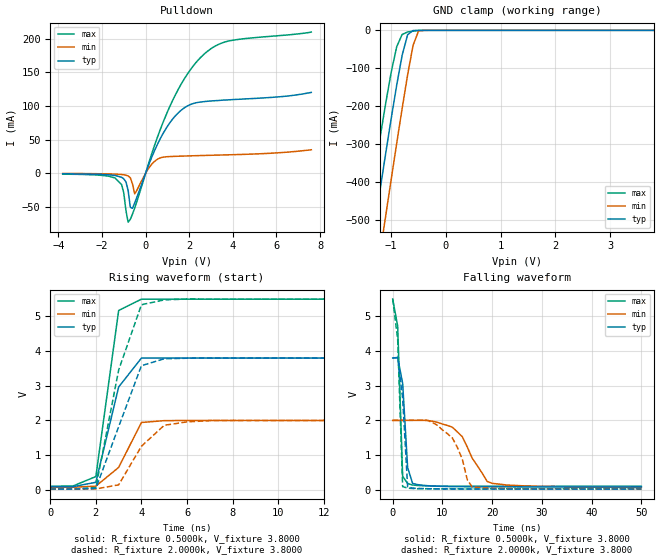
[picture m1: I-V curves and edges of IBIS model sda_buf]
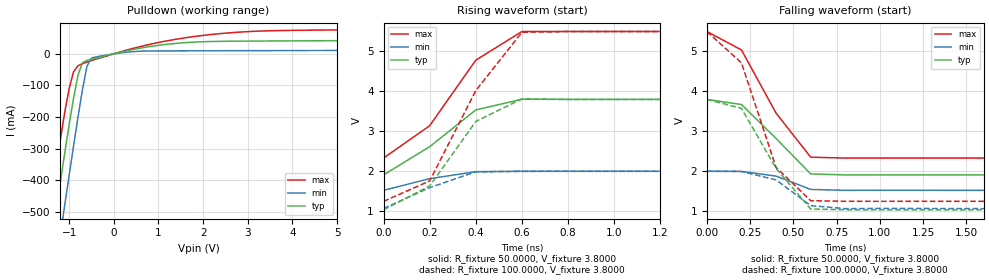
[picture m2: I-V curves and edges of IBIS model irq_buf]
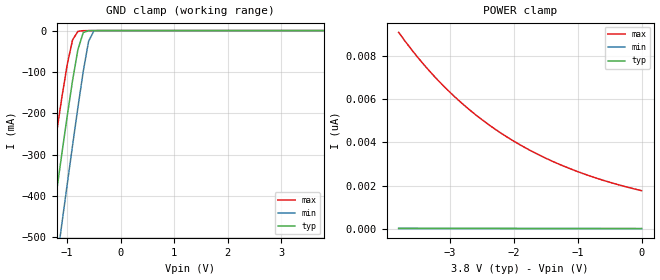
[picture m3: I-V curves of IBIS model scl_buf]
| IBIS file m41t81s.ibs created by s2ibis2 version 1.1
| North Carolina State University Electronics Research Laboratory  1995
[IBIS ver]   2.1
[File name]   m41t81s.ibs
[File Rev]   0
[Date]   August 12, 2011
[Source]   ST models
[Copyright]   ST Microelectronics Inc.
|   Component m41t81s [Package]
[Component] m41t81s
[Manufacturer]   ST Microelectronics
[Package]
| variable   typ   min   max
R_pkg   10.0000m   10.0000m   10.0000m
L_pkg   5.1000nH   4.8000nH   5.3000nH
C_pkg   0.2800pF   0.2600pF   0.2900pF
[Pin]  signal_name   model_name   R_pin   L_pin   C_pin
| N   N   dummy
| rdlowdummy   dummy
| oe   dummy   dummy
3   VBAT   NC
4   VSS   GND
5   SDAPAD   sda_buf
6   SCL   scl_buf
7   IRQB   irq_buf
8   VCC   POWER
| Models and submodels in the file (3): sda_buf (I/O_open_drain), irq_buf (Open_drain), scl_buf (Input)
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|   Model sda_buf
[Model]   sda_buf
Model_type   I/O_open_drain
Polarity   Non-Inverting
Enable   Active-High
Vinl =   1.5000V
Vinh =   2.0000V
Vmeas =   1.5000V
Cref =1.000e-10F
Rref =   0.6450k
Vref =   1.7500V
C_comp   5.3400pF   4.9000pF   5.5000pF
[Temperature Range]   27.0000   -40.0000   85.0000
[Voltage Range]   3.8000V   2.0000V   5.5000V
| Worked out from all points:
|   slope of the pulldown table from 0 to 0.57 V, typ, clamps not added: 12.7 ohm
|   GND clamp passes 1 mA (typ) near -0.60 V on its own axis
|   rising waveform, R_fixture 0.5000k, V_fixture 3.8000: 20-80 % time 888ps typ, 1.1ns min, 676ps max; typ from 0.083 V to 3.8 V
|   rising waveform, R_fixture 2.0000k, V_fixture 3.8000: 20-80 % time 1.28ns typ, 1.33ns min, 1.19ns max; typ from 0.021 V to 3.8 V
|   falling waveform, R_fixture 0.5000k, V_fixture 3.8000: 20-80 % time 918ps typ, 4.69ns min, 749ps max; typ from 3.8 V to 0.084 V
|   falling waveform, R_fixture 2.0000k, V_fixture 3.8000: 20-80 % time 1.07ns typ, 3.66ns min, 821ps max; typ from 3.8 V to 0.021 V
[Pulldown]
| voltage   I(typ)   I(min)   I(max)
-3.8V     -600uA     -200uA     -1.2mA
-1.4V     -3.13mA    -1.08mA    -6.8mA
-1.1V     -5.82mA    -1.69mA    -16.77mA
-800mV    -25.4mA    -3.87mA    -72.55mA
-700mV    -50.42mA   -6.52mA    -68.36mA
-600mV    -51.89mA   -15.66mA   -60.43mA
-500mV    -44.07mA   -30.48mA   -51.56mA
300mV     25.36mA    14.19mA    30.9mA
1V        69.82mA    24.76mA    91.21mA
2.5V      105.9mA    26.44mA    171.4mA
3.8V      109.2mA    27.56mA    196.6mA
7.6V      120.3mA    35.05mA    209.9mA
[GND_clamp]
| voltage   I(typ)   I(min)   I(max)
-3.8V     -2.967A    -3.151A    -2.807A
-1.5V     -703.8mA   -877.1mA   -557.8mA
-1.4V     -607.6mA   -779.4mA   -463.6mA
-1.3V     -512.1mA   -682.1mA   -370.7mA
-1.2V     -417.4mA   -585.2mA   -279.7mA
-1.1V     -324mA     -488.8mA   -191.9mA
-900mV    -144.9mA   -298.7mA   -43.54mA
-800mV    -65.61mA   -206.1mA   -10.92mA
-700mV    -11.59mA   -117.4mA   -4.335mA
-600mV    -529uA     -39.4mA    -1.98mA
-500mV    -33.91uA   -1.767mA   -723.6uA
3.8V      21.11pA    17.07pA    29.74nA
[Ramp]
| variable   typ   min   max
dV/dt_r   1.7910/0.8294n   0.7219/1.5223n   2.7088/0.7356n
dV/dt_f   1.7932/3.1050n   0.7044/15.8077n   2.7076/1.5825n
R_load = 50.0000
[Rising Waveform]
R_fixture = 0.5000k
V_fixture = 3.8000
V_fixture_min = 2.0000
V_fixture_max = 5.5000
| time   V(typ)   V(min)   V(max)
0s        83.25mV    69.23mV    101.4mV
1ns       88.35mV    73.11mV    109.4mV
2ns       215.8mV    104.3mV    380.3mV
3ns       2.965V     644.3mV    5.172V
4ns       3.799V     1.941V     5.5V
5ns       3.8V       1.994V     5.5V
6ns       3.8V       1.999V     5.5V
50ns      3.8V       2V         5.5V
[Rising Waveform]
R_fixture = 2.0000k
V_fixture = 3.8000
V_fixture_min = 2.0000
V_fixture_max = 5.5000
| time   V(typ)   V(min)   V(max)
0s        20.83mV    17.17mV    25.38mV
1ns       18.04mV    16.74mV    20.64mV
2ns       38.32mV    23.09mV    63.47mV
3ns       1.818V     141.4mV    3.454V
4ns       3.58V      1.254V     5.339V
5ns       3.78V      1.86V      5.479V
6ns       3.795V     1.958V     5.503V
8ns       3.8V       2V         5.499V
50ns      3.8V       2V         5.5V
[Falling Waveform]
R_fixture = 0.5000k
V_fixture = 3.8000
V_fixture_min = 2.0000
V_fixture_max = 5.5000
| time   V(typ)   V(min)   V(max)
0s        3.8V       2V         5.5V
1ns       3.807V     2.001V     4.719V
2ns       3.071V     2.001V     392mV
3ns       642mV      2.001V     179mV
4ns       183.4mV    2.001V     138.2mV
12ns      91.89mV    1.804V     103.2mV
14ns      88.72mV    1.53V      102.5mV
19ns      84.92mV    239.7mV    101.2mV
20ns      84.54mV    186.4mV    101.3mV
50ns      83.56mV    72.06mV    100.9mV
[Falling Waveform]
R_fixture = 2.0000k
V_fixture = 3.8000
V_fixture_min = 2.0000
V_fixture_max = 5.5000
| time   V(typ)   V(min)   V(max)
0s        3.8V       2V         5.5V
1ns       3.817V     2.001V     4.331V
2ns       2.636V     2.004V     92.29mV
3ns       82.17mV    2.005V     46.94mV
7ns       30.68mV    2.001V     29.97mV
12ns      23.65mV    1.494V     27.2mV
14ns      22.29mV    883.5mV    25.65mV
15ns      21.41mV    288.4mV    24.38mV
16ns      21.27mV    77.09mV    24.28mV
50ns      21.37mV    18.51mV    26.91mV
|   Model irq_buf
[Model]   irq_buf
Model_type   Open_drain
Polarity   Inverting
C_comp   5.0800pF   4.8900pF   5.2600pF
[Temperature Range]   27.0000   -40.0000   85.0000
[Voltage Range]   3.8000V   2.0000V   5.5000V
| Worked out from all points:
|   slope of the pulldown table from 0 to 0.57 V, typ, clamps not added: 32.6 ohm
|   rising waveform, R_fixture 50.0000, V_fixture 3.8000: 20-80 % time 268ps typ, 237ps min, 267ps max; typ from 1.91 V to 3.8 V
|   rising waveform, R_fixture 100.0000, V_fixture 3.8000: 20-80 % time 214ps typ, 241ps min, 256ps max; typ from 1.04 V to 3.8 V
|   falling waveform, R_fixture 50.0000, V_fixture 3.8000: 20-80 % time 262ps typ, 200ps min, 267ps max; typ from 3.8 V to 1.91 V
|   falling waveform, R_fixture 100.0000, V_fixture 3.8000: 20-80 % time 251ps typ, 193ps min, 195ps max; typ from 3.8 V to 1.04 V
[Pulldown]
| voltage   I(typ)   I(min)   I(max)
-3.8V     -2.956A    -3.143A    -2.795A
-1.7V     -888.1mA   -1.065A    -738.1mA
-1.4V     -598.7mA   -771.9mA   -454.4mA
-1.1V     -316.4mA   -481.6mA   -187.2mA
-900mV    -140.6mA   -292.1mA   -56.91mA
-800mV    -67.1mA    -200.2mA   -37.9mA
-700mV    -27.98mA   -112.9mA   -31.15mA
-600mV    -20.85mA   -39.87mA   -25.89mA
-500mV    -17.44mA   -13.08mA   -21.24mA
900mV     25.04mA    9.181mA    32.91mA
2.4V      39.61mA    9.862mA    64.32mA
7.6V      45.25mA    13.15mA    78.93mA
[Ramp]
| variable   typ   min   max
dV/dt_r   1.1348/0.2108n   0.2862/0.1639n   1.9019/0.2327n
dV/dt_f   1.1354/0.2151n   0.2866/0.1466n   1.9015/0.2396n
R_load = 50.0000
[Rising Waveform]
R_fixture = 50.0000
V_fixture = 3.8000
V_fixture_min = 2.0000
V_fixture_max = 5.5000
| time   V(typ)   V(min)   V(max)
0s        1.909V     1.523V     2.33V
200ps     2.616V     1.815V     3.14V
400ps     3.536V     1.99V      4.783V
600ps     3.804V     2V         5.5V
10ns      3.8V       2V         5.5V
[Rising Waveform]
R_fixture = 100.0000
V_fixture = 3.8000
V_fixture_min = 2.0000
V_fixture_max = 5.5000
| time   V(typ)   V(min)   V(max)
0s        1.037V     1.068V     1.247V
200ps     1.632V     1.59V      1.758V
400ps     3.248V     1.988V     4.02V
600ps     3.814V     1.998V     5.481V
800ps     3.799V     2V         5.5V
10ns      3.8V       2V         5.5V
[Falling Waveform]
R_fixture = 50.0000
V_fixture = 3.8000
V_fixture_min = 2.0000
V_fixture_max = 5.5000
| time   V(typ)   V(min)   V(max)
0s        3.8V       2V         5.5V
200ps     3.67V      1.997V     5.038V
400ps     2.821V     1.879V     3.455V
600ps     1.934V     1.545V     2.353V
800ps     1.908V     1.522V     2.331V
10ns      1.908V     1.522V     2.331V
[Falling Waveform]
R_fixture = 100.0000
V_fixture = 3.8000
V_fixture_min = 2.0000
V_fixture_max = 5.5000
| time   V(typ)   V(min)   V(max)
0s        3.8V       2V         5.5V
200ps     3.575V     1.994V     4.715V
400ps     2.071V     1.784V     2.095V
600ps     1.055V     1.14V      1.263V
800ps     1.036V     1.064V     1.247V
10ns      1.036V     1.065V     1.246V
|   Model scl_buf
[Model]   scl_buf
Model_type   Input
Vinl =   0.3000V
Vinh =   0.7000V
C_comp   4.7600pF   4.5300pF   4.7600pF
[Temperature Range]   27.0000   -40.0000   85.0000
[Voltage Range]   3.8000V   2.0000V   5.5000V
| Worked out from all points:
|   GND clamp passes 1 mA (typ) near -0.62 V on its own axis
[GND_clamp]
| voltage   I(typ)   I(min)   I(max)
-3.8V     -2.938A    -3.129A    -2.774A
-1.5V     -676.3mA   -855.5mA   -525mA
-1.4V     -580.3mA   -757.9mA   -431.1mA
-1.3V     -485mA     -660.7mA   -338.6mA
-1.1V     -297.6mA   -467.6mA   -161.5mA
-1V       -207mA     -372.2mA   -82.33mA
-900mV    -120.9mA   -278.1mA   -22.58mA
-800mV    -45.94mA   -186.1mA   -1.937mA
-700mV    -4.748mA   -98.85mA   -206.1uA
-600mV    -123.9uA   -25.82mA   -66.48uA
-500mV    -3.317uA   -623.5uA   -23.23uA
3.8V      9.231pA    9.491pA    930.4pA
[POWER_clamp]
| voltage   I(typ)   I(min)   I(max)
-3.8V     18.85pA    14.49pA    9.096nA
-3.6V     18.32pA    13.99pA    8.304nA
-3.4V     17.79pA    13.49pA    7.582nA
-3.2V     17.26pA    12.99pA    6.925nA
-3V       16.74pA    12.49pA    6.328nA
-2.6V     15.71pA    11.49pA    5.289nA
-2.2V     14.69pA    10.49pA    4.431nA
-2V       14.18pA    9.991pA    4.059nA
-1.7V     13.43pA    9.242pA    3.563nA
-1.2V     12.18pA    7.993pA    2.879nA
-600mV    10.7pA     6.494pA    2.245nA
0V        9.231pA    4.996pA    1.765nA
